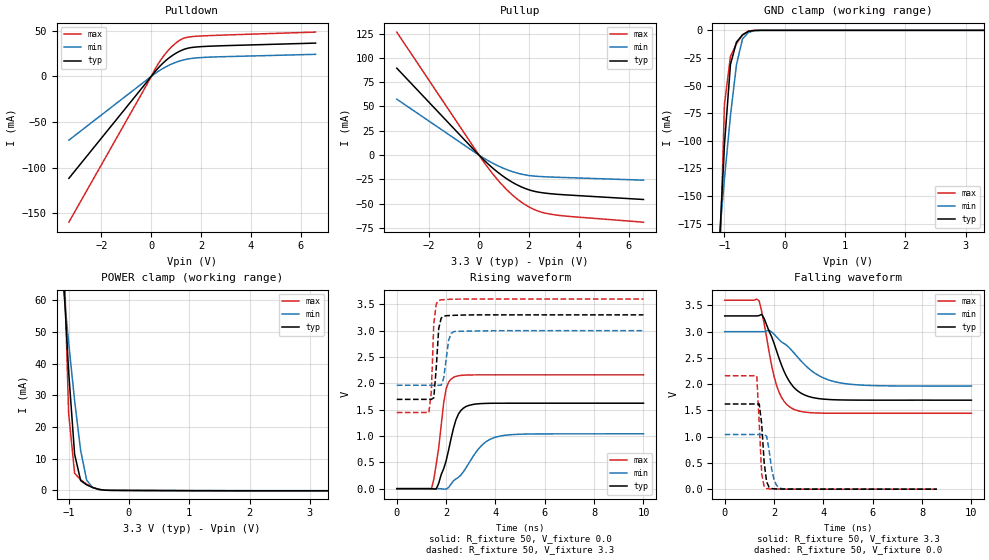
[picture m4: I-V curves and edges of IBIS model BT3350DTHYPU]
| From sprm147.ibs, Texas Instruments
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[Model]   BT3350DTHYPU
Model_type   I/O
Vinh = 2.00
Vinl = 0.80
Enable   Active-Low
Polarity   Non-Inverting
| signals   A, GZ, Y
Vmeas = 1.5
|   typ   min   max
C_comp   1.3098752p   1.2583746p   1.386713p
|   typ   min   max
[Temperature Range]   25   -40   125
|   typ   min   max
[Voltage Range]   3.30V   3.00V   3.60V
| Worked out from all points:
|   slope of the pulldown table from 0 to 0.495 V, typ, clamps not added: 32.6 ohm
|   slope of the pullup table from 0 to 0.495 V, typ, clamps not added: 40.8 ohm
|   GND clamp passes 1 mA (typ) near -0.60 V on its own axis
|   POWER clamp passes 1 mA (typ) near -0.61 V on its own axis
|   rising waveform, R_fixture 50, V_fixture 0.0: 20-80 % time 540ps typ, 994ps min, 349ps max; typ from 0 V to 1.62 V
|   falling waveform, R_fixture 50, V_fixture 3.3: 20-80 % time 847ps typ, 1.44ns min, 586ps max; typ from 3.3 V to 1.7 V
|   rising waveform, R_fixture 50, V_fixture 3.3: 20-80 % time 140ps typ, 173ps min, 106ps max; typ from 1.7 V to 3.3 V
|   falling waveform, R_fixture 50, V_fixture 0.0: 20-80 % time 164ps typ, 223ps min, 138ps max; typ from 1.62 V to 0 V
[Pulldown]
|   Voltage   I(typ)   I(min)   I(max)
-3.3V     -111.9mA   -69.95mA   -160.1mA
-200mV    -7.006mA   -4.259mA   -10.31mA
200mV     6.741mA    4.038mA    10.03mA
400mV     12.65mA    7.622mA    18.63mA
600mV     17.74mA    10.75mA    25.92mA
1V        25.63mA    15.66mA    36.92mA
1.3V      29.62mA    18.2mA     41.96mA
1.7V      32.11mA    20.12mA    43.97mA
6.6V      36.69mA    24.35mA    48.79mA
[GND_clamp]
|   Voltage   I(typ)   I(min)   I(max)
-3.3V     -3.122A    -1.743A    -6.724A
-1.1V     -211.8mA   -197.5mA   -255.4mA
-1V       -104mA     -134.8mA   -67.2mA
-900mV    -30.82mA   -77.2mA    -23.58mA
-800mV    -10.62mA   -31.04mA   -12.09mA
-700mV    -4.144mA   -7.761mA   -4.059mA
-600mV    -907.7uA   -1.845mA   -578.7uA
-500mV    -93.1uA    -343.8uA   -34.38uA
-400mV    -5.844uA   -44.19uA   -1.039uA
3.3V      222pA      7.672uA    0A
[Pullup]
|   Voltage   I(typ)   I(min)   I(max)
-3.3V     89.4mA     57.53mA    126.5mA
300mV     -7.585mA   -4.745mA   -10.94mA
700mV     -16.55mA   -10.25mA   -24mA
1V        -22.37mA   -13.74mA   -32.59mA
1.6V      -31.52mA   -18.93mA   -46.5mA
1.9V      -34.77mA   -20.57mA   -51.74mA
2.2V      -37.1mA    -21.57mA   -55.78mA
2.5V      -38.56mA   -22.09mA   -58.6mA
2.9V      -39.76mA   -22.56mA   -60.85mA
3.7V      -41.23mA   -23.28mA   -63.23mA
6.6V      -45.64mA   -25.79mA   -68.98mA
[POWER_clamp]
|   Voltage   I(typ)   I(min)   I(max)
-3.3V     979.7mA    549.5mA    2.105A
-1.1V     72.52mA    66.76mA    89.69mA
-1V       37.74mA    46.91mA    24.47mA
-900mV    11.42mA    28.34mA    5.41mA
-800mV    3.12mA     12.58mA    3.377mA
-700mV    1.751mA    3.26mA     2mA
-600mV    921.2uA    893.4uA    960uA
-500mV    358.7uA    314.9uA    300.9uA
-400mV    86.67uA    81.35uA    67.3uA
3.3V      -100.1uA   -62.4uA    -157uA
[Ramp]
|   I(typ)   I(min)   I(max)
dV/dt_r   0.973/0.538n   0.625/0.984n   1.296/0.345n
dV/dt_f   0.963/0.841n   0.622/1.443n   1.292/0.584n
[Rising Waveform]
R_fixture = 50
V_fixture = 0.0
|  pu_on
|  TIME   V(typ)   V(min)   V(max)
0s        18nV       187nV      1nV
1.4ns     396.2uV    -3.671uV   -8.727mV
1.6ns     -5.678mV   -904nV     467.3mV
2ns       528.8mV    -8.769mV   1.897V
2.3ns     1.15V      149.2mV    2.114V
2.5ns     1.417V     215.9mV    2.144V
2.8ns     1.559V     389.1mV    2.157V
3.4ns     1.615V     800.6mV    2.161V
4.1ns     1.622V     989.2mV    2.161V
10ns      1.622V     1.041V     2.161V
[Falling Waveform]
R_fixture = 50
V_fixture = 3.3
V_fixture_min = 3.0
V_fixture_max = 3.6
|  pd_on
|  TIME   V(typ)   V(min)   V(max)
0s        3.3V       3V         3.6V
1.4ns     3.307V     3V         3.585V
1.6ns     3.25V      3V         3.153V
1.9ns     2.907V     2.995V     2.362V
2.1ns     2.636V     2.902V     1.981V
2.4ns     2.251V     2.776V     1.677V
2.8ns     1.94V      2.6V       1.522V
3.6ns     1.742V     2.227V     1.454V
4.6ns     1.701V     2.032V     1.446V
10ns      1.695V     1.963V     1.446V
[Rising Waveform]
R_fixture = 50
V_fixture = 3.3
V_fixture_min = 3.0
V_fixture_max = 3.6
|  pd_off
|  TIME   V(typ)   V(min)   V(max)
0s        1.695V     1.963V     1.446V
1.3ns     1.695V     1.963V     1.444V
1.4ns     1.695V     1.963V     1.833V
1.5ns     1.725V     1.963V     3.133V
1.6ns     2.293V     1.964V     3.51V
1.7ns     3.042V     1.962V     3.572V
1.9ns     3.275V     2.097V     3.588V
2.1ns     3.287V     2.816V     3.594V
2.3ns     3.291V     2.979V     3.598V
10ns      3.3V       3V         3.6V
[Falling Waveform]
R_fixture = 50
V_fixture = 0.0
|  pu_off
|  TIME   V(typ)   V(min)   V(max)
0s        1.622V     1.041V     2.161V
1.3ns     1.622V     1.041V     2.159V
1.4ns     1.623V     1.041V     1.246V
1.5ns     1.242V     1.04V      288.2mV
1.6ns     502.9mV    1.043V     52.38mV
1.7ns     139.9mV    1.008V     11.88mV
1.9ns     12.38mV    394.6mV    3.148mV
2ns       6.342mV    183.8mV    2.395mV
2.3ns     2.637mV    11.11mV    1.062mV
8.6ns     1.017uV    2.394uV    910nV
